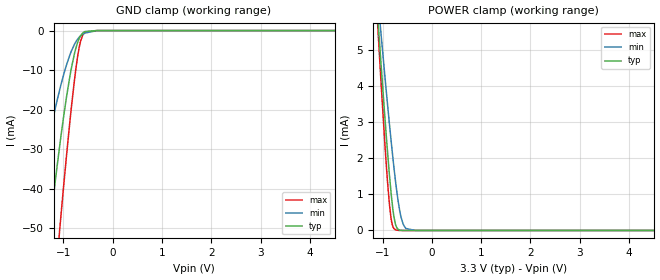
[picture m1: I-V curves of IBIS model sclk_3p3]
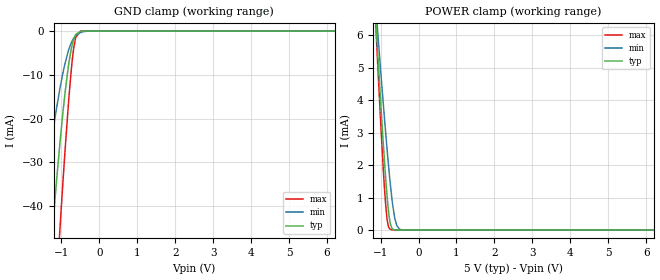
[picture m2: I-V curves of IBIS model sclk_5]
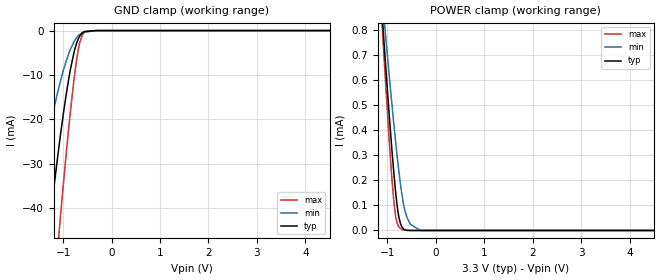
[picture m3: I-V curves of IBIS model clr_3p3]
|Texas Instruments Incorporated
| DAC8771 Single-Channel, 16-Bit Voltage and Current Output Digital-to-Analog
| Converter with Adaptive Power Management
| Marketing part#   Digital Voltage Range   Package-type   #pins
| DAC8771   2.7V-5.5V   VQFN   48
[IBIS Ver]   4.1
[File name]   dac8771.ibs
[File Rev]   1.0
[Date]   11/18/2016
[Source]
| Texas Instruments Incorporated.
| Analog-eLab Design Center, HPA
| 12500 TI Blvd
| Dallas, TX -75243
[Notes]   Revision History:
| Rev 1.0: 11/18/2016
| - Initial version of the model
| - Model generated from simulations in SPECTRE
| - Model matched to SPICE simulation
| - C_comp although listed in numerical order of value are
|   obtained from varying PVT conditions. For PVT conditions for
|   each specific value refer the buffer description under
|   respective [Model]. IBIS model user is responsible for using
|   appropriate C_comp to simulate for Signal Integrity.
|*EXCEPTION:   *
|* -For model sdo pullup and pulldown IV tables does not pass through 0   *
|*  because of because of driver switch(MP0-3,MP10-17,MN3-6,MN11-14)   *
|*  arrangement.   *
|* -For model alarm,pulldown IV tables does not pass through 0 because   *
|*  of because of pulldown transistor(MN0) attached to pad.   *
[Disclaimer]
| This model is designed as an aid for customers of Texas Instruments.
| TI and its licensors and suppliers make no warranties, either expressed
| or implied, with respect to this  model, including the warranties of
| merchantability or fitness for a particular purpose. The model is
| provided solely on an "as is" basis. The entire risk as to its quality
| and performance is with the customer.
[Copyright]
(C) Copyright 2016 Texas Instruments Incorporated.All rights reserved.
|   DAC8771
[Component]   DAC8771
[Manufacturer]   TI
[Package]   |48 VQFN
|   typ   min   max
R_pkg   0.1   0.08   0.12
L_pkg   1.0nH   0.8nH   1.2nH
C_pkg   0.2pF   0.16pF   0.24pF
[Pin]  signal_name   model_name   R_pin   L_pin   C_pin
1   NC   nc   NA   NA   NA
2   AVDD   power   NA   NA   NA
3   GND   gnd   NA   NA   NA
4   REFOUT   nc   NA   NA   NA
5   REFIN   nc   NA   NA   NA
6   DVDD_EN   nc   NA   NA   NA
7   DVDD   power   NA   NA   NA
8   NC   nc   NA   NA   NA
9   GND   gnd   NA   NA   NA
10   NC   nc   NA   NA   NA
11   VNEG_IN   power   NA   NA   NA
12   NC   nc   NA   NA   NA
13   NC   nc   NA   NA   NA
14   PVDD   power   NA   NA   NA
15   LP   nc   NA   NA   NA
16   PVSS   gnd   NA   NA   NA
17   LN   nc   NA   NA   NA
18   GND   gnd   NA   NA   NA
19   NC   nc   NA   NA   NA
20   GND   gnd   NA   NA   NA
21   NC   nc   NA   NA   NA
22   BOOST   nc   NA   NA   NA
23   VPOS_IN   power   NA   NA   NA
24   NC   nc   NA   NA   NA
25   VOUT   power   NA   NA   NA
26   IOUT   nc   NA   NA   NA
27   VNEG_IN   power   NA   NA   NA
28   GND   gnd   NA   NA   NA
29   VSENSEP   nc   NA   NA   NA
30   VSENSEN   nc   NA   NA   NA
31   CCOMP   nc   NA   NA   NA
32   HART_IN   nc   NA   NA   NA
33   RSET   nc   NA   NA   NA
34   RSET_SENSE   nc   NA   NA   NA
35   RSET_EN   nc   NA   NA   NA
36   NC   nc   NA   NA   NA
37   NC   nc   NA   NA   NA
38   SDO   sdo   NA   NA   NA
39   SDIN   sclk   NA   NA   NA
40   SCLK   sclk   NA   NA   NA
41   _SYNC   sclk   NA   NA   NA
42   _LDAC   clr   NA   NA   NA
43   CLR   clr   NA   NA   NA
44   _RESET   sclk   NA   NA   NA
45   _ALARM   alarm   NA   NA   NA
46   NC   nc   NA   NA   NA
47   NC   nc   NA   NA   NA
48   NC   nc   NA   NA   NA
|   Model Selectors
[Model Selector] sclk
sclk_3p3   3.3V  digital Input
sclk_5   5.0V  digital Input
[Model Selector] clr
clr_3p3   3.3V  digital Input
clr_5   5.0V  digital Input
[Model Selector] sdo
sdo_3p3   3.3V  digital Output
sdo_5   5.0V  digital Output
[Model Selector] alarm
alarm_3p3   3.3V  digital Open_drain
alarm_5   5.0V  digital Open_drain
| Models and submodels in the file (8): sclk_3p3 (Input), sclk_5 (Input), clr_3p3 (Input), clr_5 (Input), sdo_3p3 (Output), sdo_5 (Output), alarm_3p3 (Open_drain), alarm_5 (Open_drain)
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|   sclk_3p3 Model
[Model]   sclk_3p3
Model_type   Input
Vinl = 0.6
Vinh = 2
|   typ   min   max
|   (nom PVT)   (fast PVT)   (slow PVT)
C_comp   1.437e-12   1.404e-12   1.437e-12
| Where nom  PVT is Nominal Process, 3.3V, 27C
|   Fast PVT is Strong Process,  3.9V, -40C
|   Slow PVT is Weak Process,   2.7V, 150C
[Voltage Range]   3.3   2.7   3.9
|Junction Temperature
[Temperature Range]   27   150   -40
[Power Clamp Reference]   3.3   2.7   3.9
[GND Clamp Reference]   0   0   0
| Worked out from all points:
|   GND clamp passes 1 mA (typ) near -0.63 V on its own axis
|   POWER clamp passes 1 mA (typ) near -0.82 V on its own axis
[GND Clamp]
|   Voltage   I(typ)   I(min)   I(max)
-3.3V     -310.5mA   -204.7mA   -387.4mA
-1.621V   -90.38mA   -50.03mA   -131.4mA
-1.278V   -50.2mA    -26.38mA   -79.81mA
-1.129V   -34.44mA   -17.75mA   -58.05mA
-1.053V   -27.03mA   -13.86mA   -47.33mA
-940.5mV  -17.12mA   -8.842mA   -32.16mA
-841.5mV  -9.752mA   -5.297mA   -19.86mA
-749.4mV  -4.558mA   -2.899mA   -9.94mA
-679.8mV  -1.999mA   -1.699mA   -4.273mA
-603.9mV  -566.9uA   -903.3uA   -1.05mA
-562.2mV  -236.6uA   -630.5uA   -397.2uA
6.6V      0A         0A         0A
[POWER Clamp]
|   Voltage   I(typ)   I(min)   I(max)
-3.3V     52.59mA    42.53mA    61.55mA
-1.172V   7.402mA    7.612mA    7.43mA
-1.046V   4.886mA    5.658mA    4.431mA
-1.03V    4.572mA    5.412mA    4.061mA
-920.7mV  2.543mA    3.796mA    1.738mA
-862.5mV  1.561mA    2.969mA    747.8uA
-810.6mV  815.5uA    2.266mA    203.2uA
-742.5mV  193.2uA    1.421mA    20.97uA
-653.4mV  10.21uA    554uA      1.679uA
-581.1mV  806.4nA    166.8uA    202.6nA
-328.2mV  0A         293.3nA    0A
6.6V      0A         0A         0A
|   sclk_5 Model
[Model]   sclk_5
Model_type   Input
Vinl = 0.8
Vinh = 2
|   typ   min   max
|   (nom PVT)   (fast PVT)   (slow PVT)
C_comp   1.404e-12   1.371e-12   1.404e-12
| Where nom  PVT is Nominal Process, 5V, 27C
|   Fast PVT is Strong Process,  5.5V, -40C
|   Slow PVT is Weak Process,   4.5V, 150C
[Voltage Range]   5   4.5   5.5
|Junction Temperature
[Temperature Range]   27   150   -40
[Power Clamp Reference]   5   4.5   5.5
[GND Clamp Reference]   0   0   0
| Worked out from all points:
|   GND clamp passes 1 mA (typ) near -0.64 V on its own axis
|   POWER clamp passes 1 mA (typ) near -0.83 V on its own axis
[GND Clamp]
|   Voltage   I(typ)   I(min)   I(max)
-5V       -539.4mA   -387mA     -645.4mA
-1.573V   -84.43mA   -46.39mA   -124mA
-1.328V   -55.61mA   -29.42mA   -87.05mA
-1.17V    -38.49mA   -19.93mA   -63.79mA
-1.13V    -34.41mA   -17.73mA   -58.03mA
-1.03V    -24.76mA   -12.69mA   -43.96mA
-905mV    -14.17mA   -7.399mA   -27.4mA
-800mV    -7.083mA   -4.055mA   -14.98mA
-675.5mV  -1.837mA   -1.617mA   -3.907mA
-620mV    -744.7uA   -1.02mA    -1.43mA
-500mV    -51.05uA   -350.3uA   -75.3uA
10V       0A         0A         0A
[POWER Clamp]
|   Voltage   I(typ)   I(min)   I(max)
-5V       89.26mA    70.95mA    105.4mA
-1.234V   8.607mA    8.542mA    8.878mA
-1.1V     5.918mA    6.461mA    5.66mA
-1.079V   5.493mA    6.13mA     5.154mA
-936.5mV  2.794mA    4mA        2.016mA
-869.5mV  1.646mA    3.042mA    826.4uA
-824mV    968.3uA    2.42mA     289.9uA
-743mV    187.2uA    1.406mA    20.23uA
-625mV    3.521uA    354.2uA    722.4nA
-572mV    557.3nA    134uA      144.3nA
-437mV    0A         5.044uA    0A
10V       0A         0A         0A
|   clr_3p3 Model
[Model]   clr_3p3
Model_type   Input
Vinl = 0.6
Vinh = 2
|   typ   min   max
|   (nom PVT)   (fast PVT)   (slow PVT)
C_comp   8.232e-13   7.943e-13   8.537e-13
| Where nom  PVT is Nominal Process, 3.3V, 27C
|   Fast PVT is Strong Process,  3.9V, -40C
|   Slow PVT is Weak Process,   2.7V, 150C
[Voltage Range]   3.3   2.7   3.9
|Junction Temperature
[Temperature Range]   27   150   -40
[Power Clamp Reference]   3.3   2.7   3.9
[GND Clamp Reference]   0   0   0
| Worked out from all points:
|   GND clamp passes 1 mA (typ) near -0.64 V on its own axis
|   POWER clamp passes 1 mA (typ) near -1.16 V on its own axis
[GND Clamp]
|   Voltage   I(typ)   I(min)   I(max)
-3.3V     -273mA     -179.2mA   -340.5mA
-1.815V   -100.2mA   -56.11mA   -141.6mA
-1.623V   -79.17mA   -42.92mA   -115.9mA
-1.333V   -48.97mA   -25.1mA    -77.39mA
-1.283V   -44.05mA   -22.34mA   -70.83mA
-1.132V   -29.99mA   -14.73mA   -51.36mA
-1.059V   -23.76mA   -11.49mA   -42.29mA
-848.1mV  -8.582mA   -4.113mA   -17.91mA
-759mV    -4.153mA   -2.151mA   -9.426mA
-686.4mV  -1.8mA     -1.128mA   -4.143mA
-558.3mV  -193.9uA   -319.9uA   -324.4uA
6.6V      0A         0A         0A
[POWER Clamp]
|   Voltage   I(typ)   I(min)   I(max)
-3.3V     7.449mA    6.092mA    8.646mA
-1.189V   1.084mA    1.111mA    1.087mA
-1.058V   715.6uA    821.6uA    652uA
-1.046V   684.3uA    796.9uA    615.4uA
-933.9mV  388.1uA    559.2uA    277.5uA
-864.6mV  223.9uA    419.9uA    111.2uA
-821.7mV  137.5uA    338.3uA    47.52uA
-778.8mV  71.28uA    261.9uA    19.5uA
-705.3mV  15.89uA    149.8uA    4.825uA
-594.6mV  695.1nA    50.99uA    297.6nA
-328.2mV  0A         641.2nA    0A
6.6V      0A         0A         0A
